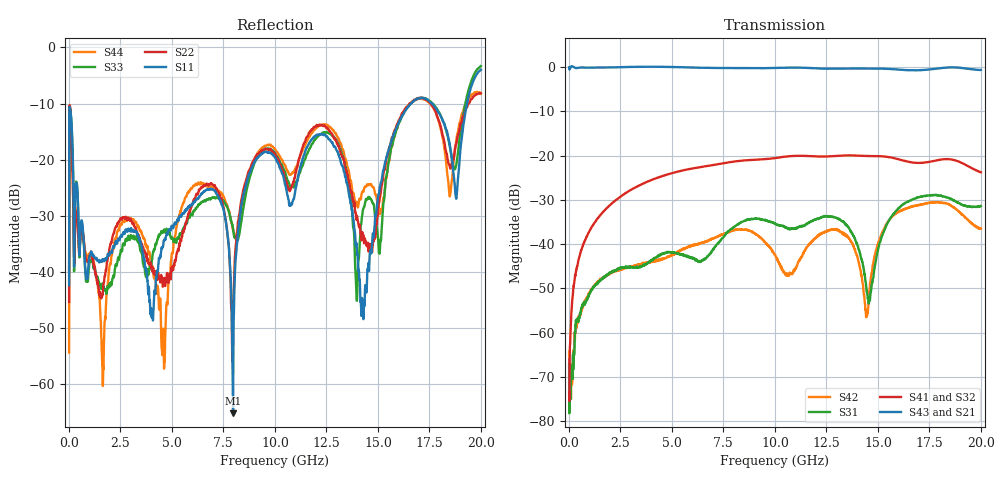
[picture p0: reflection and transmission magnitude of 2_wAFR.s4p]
!Keysight Technologies,N5225A,MY51451420,A.10.40.12
!Date: Tuesday, October 13, 2015 09:45:15
!Correction: S11(Full 4 Port(1,2,3,4))
!S12(Full 4 Port(1,2,3,4))
!S13(Full 4 Port(1,2,3,4))
!S14(Full 4 Port(1,2,3,4))
!S21(Full 4 Port(1,2,3,4))
!S22(Full 4 Port(1,2,3,4))
!S23(Full 4 Port(1,2,3,4))
!S24(Full 4 Port(1,2,3,4))
!S31(Full 4 Port(1,2,3,4))
!S32(Full 4 Port(1,2,3,4))
!S33(Full 4 Port(1,2,3,4))
!S34(Full 4 Port(1,2,3,4))
!S41(Full 4 Port(1,2,3,4))
!S42(Full 4 Port(1,2,3,4))
!S43(Full 4 Port(1,2,3,4))
!S44(Full 4 Port(1,2,3,4))
!S4P File: Measurements: <S11,S12,S13,S14>,
!<S21,S22,S23,S24>,
!<S31,S32,S33,S34>,
!<S41,S42,S43,S44>:
# Hz S  dB  R 50
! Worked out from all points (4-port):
!   2000 points, 10 MHz to 20 GHz, reference 50 ohm
!   strongest paths, dB at 10 MHz, 5.01 GHz, 10.01 GHz, 15.01 GHz, 20 GHz:
!     S43: -0.1, 0.0, -0.2, -0.4, -0.7
!     S21: 0.0, 0.0, -0.2, -0.4, -0.6
!     S41: -73.5, -24.0, -20.6, -20.2, -23.8
!     S32: -74.5, -24.0, -20.6, -20.2, -23.8
!     S31: -67.3, -41.9, -35.4, -41.2, -31.4
!     S42: -64.3, -42.5, -42.4, -39.8, -36.5
!   lowest |S11| = -65.1 dB at 7.97 GHz (marker M1), VSWR 1.00, Z = 50 + j0.0551 ohm
!   |S11| at or under -10 dB: start of sweep to 16.62 GHz; 17.62 GHz to 19.33 GHz (1.706 GHz wide, 9.24 % of centre)
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1e7  -42.34 -35.6  -0.03 0.3  -65.45 23.3  -64.48 106.9
     -0.03 0.5  -45.35 178.1  -81.71 157.3  -61.18 106.5
     -67.27 150.6  -74.49 155.1  -39.79 -15.9  -0.07 0.6
     -73.46 101.2  -64.30 102.5  -0.08 0.2  -54.33 -175.4
1.34e9  -37.47 -55.2  -0.15 7.6  -49.04 64.3  -34.56 97.2
        -0.16 7.6  -41.15 3.8  -34.53 97.1  -48.75 120.4
        -49.02 64.7  -34.55 97.3  -41.04 -36.0  -0.17 7.7
        -34.56 97.3  -48.81 120.2  -0.16 7.7  -40.56 40.1
6.98e9  -25.30 -16.6  -0.22 42.2  -41.35 -15.9  -22.17 132.6
        -0.23 42.4  -24.51 -85.2  -22.16 132.4  -38.77 -58.1
        -41.33 -16.1  -22.16 132.3  -26.80 -7.7  -0.24 42.6
        -22.17 132.8  -38.78 -57.8  -0.22 42.7  -25.09 -94.0
7.97e9  -65.14 94.4  -0.24 44.3  -36.27 -57.9  -21.39 134.6
        -0.24 44.5  -48.38 115.6  -21.36 134.1  -36.92 -46.0
        -36.30 -57.8  -21.38 134.0  -32.40 -91.6  -0.25 44.8
        -21.40 134.8  -36.95 -45.6  -0.24 44.9  -32.44 6.3
9.18e9  -19.61 108.8  -0.27 48.0  -34.25 -124.9  -20.91 137.9
        -0.28 48.3  -18.97 165.7  -20.89 137.1  -38.09 -52.1
        -34.28 -124.7  -20.90 137.0  -19.40 117.1  -0.29 48.6
        -20.92 138.1  -38.13 -51.8  -0.28 48.7  -18.69 158.0
1.426e10  -45.82 -90.4  -0.36 80.2  -44.35 173.2  -20.07 171.4
          -0.35 80.7  -33.63 -123.8  -20.06 170.4  -48.87 126.1
          -44.18 173.7  -20.07 170.3  -29.25 26.7  -0.37 81.1
          -20.07 171.9  -48.95 128.6  -0.37 81.4  -25.55 -85.3
2e10  -3.98 -97.0  -0.56 122.1  -31.41 -32.7  -23.77 -149.3
      -0.57 122.7  -8.15 -142.1  -23.83 -150.6  -36.39 -96.9
      -31.43 -32.8  -23.81 -151.0  -3.35 -93.0  -0.66 123.4
      -23.79 -148.7  -36.50 -97.3  -0.65 123.7  -8.29 -146.9
